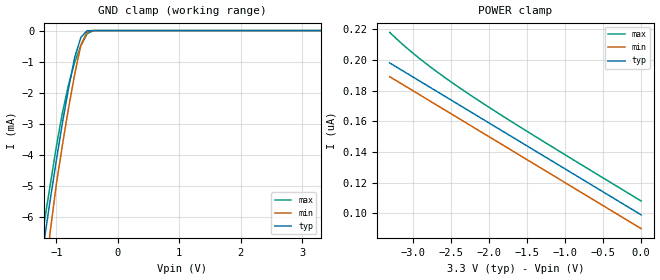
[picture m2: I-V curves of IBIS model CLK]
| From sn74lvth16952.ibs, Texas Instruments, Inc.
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|   LVTH16952 CLOCK
[Model]   CLK
|Signals
Model_type  Input
Polarity   Non-Inverting
Vinl = 0.8V
Vinh = 2.0V
| variable   typ   min   max
C_comp   4p   NA   NA
[Temperature Range]   50   100   0
[Voltage range]   3.3   3   3.6
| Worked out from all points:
|   GND clamp passes 1 mA (typ) near -0.71 V on its own axis
|Process range|   weak   strong
[GND Clamp]
|   50C:3.3V:   100C:3V:weak   0C:3.6V:strong
|   Voltage   I(typ)   I(min)   I(max)
-3.3V     -82.56mA   -87.25mA   -78mA
-1.3V     -8.397mA   -11.24mA   -7.565mA
-1.2V     -6.802mA   -8.589mA   -6.234mA
-1.1V     -5.466mA   -6.489mA   -4.985mA
-1V       -4.185mA   -4.956mA   -3.74mA
-900mV    -2.972mA   -3.679mA   -2.645mA
-800mV    -1.847mA   -2.485mA   -1.736mA
-700mV    -850.9uA   -1.396mA   -1.012mA
-600mV    -217.5uA   -464.6uA   -483.6uA
-500mV    -3.507uA   -47.7uA    -105.5uA
-400mV    -109.5nA   -2.391uA   -790.3nA
3.3V      99nA       99.03nA    99.02nA
[POWER Clamp]
|   50C:3.3V:   100C:3V:weak   0C:3.6V:strong
|   Voltage   I(typ)   I(min)   I(max)
-3.3V     198nA      189.1nA    217.9nA
-3.1V     192nA      183.1nA    208.8nA
-2.9V     186nA      177.1nA    200.5nA
-2.6V     177nA      168nA      189.3nA
-2.3V     168nA      159nA      179nA
-1.5V     144nA      135nA      153.5nA
0V        99nA       90.03nA    108nA
